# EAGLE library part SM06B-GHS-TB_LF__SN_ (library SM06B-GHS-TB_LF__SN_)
GH 1.25mm header side entry 6 way JST GH Series, 1.25mm Pitch 6 Way Right Angle PCB Header, Solder Termination, 1A Source: Datasheet
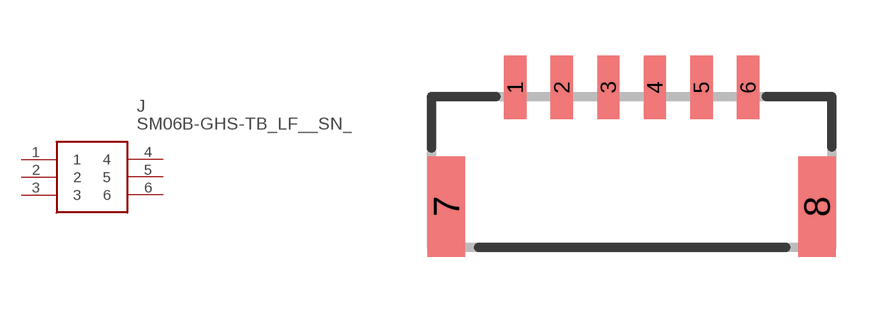
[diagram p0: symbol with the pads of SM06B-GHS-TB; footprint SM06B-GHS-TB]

Designator prefix J

## SM06B-GHS-TB_LF__SN_ (Arrow_Part_Number: SM06B-GHS-TB(LF)(SN); Arrow_Price-Stock: https://www.arrow.com/en/products/sm06b-ghs-tb-lf-sn/jst-manufacturing; Description: GH 1.25mm header side entry 6 way JST GH Series, 1.25mm Pitch 6 Way Right Angle PCB Header, Solder Termination, 1A; Height: mm; Manufacturer_Name: JST (JAPAN SOLDERLESS TERMINALS); Manufacturer_Part_Number: SM06B-GHS-TB(LF)(SN); Mouser_Part_Number: N/A; Mouser_Price-Stock: https://www.mouser.co.uk/ProductDetail/JST-Commercial/SM06B-GHS-TBLFSN?qs=QpmGXVUTftFzTQe43vH9Ig%3D%3D)  [SM06B-GHS-TB]
1  1
2  2
3  3
4  4
5  5
6  6

## Footprint SM06B-GHS-TB (pad centres in mm)
SM06B-GHS-TB
smd 0.6 x 1.7: 1 2.25,4.3; 2 3.5,4.3; 3 4.75,4.3; 4 6,4.3; 5 7.25,4.3; 6 8.5,4.3
smd 1 x 2.7: 7 0.4,1.1; 8 10.35,1.1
